| IBIS file bga289.ibs generated by Viper version: 2021.04.12
[IBIS Ver]   5.0
[Comment Char]   |_char
[File Name]   imxrt1180_c0_bga289_consmr.ibs
[File Rev]   1
[Date]   Mon Sep 20 18:29:29 2021
[Source]   NXP Viper 2021.04.12
[Notes]
[Disclaimer] IMPORTANT NOTICE
  This information is provided on an AS IS basis and without warranty.
  IN NO EVENT SHALL NXP BE LIABLE FOR INCIDENTAL OR CONSEQUENTIAL
  DAMAGES ARISING FROM USE OF THIS INFORMATION. THIS DISCLAIMER OF
  WARRANTY EXTENDS TO THE USER OF THE INFORMATION, AND TO THEIR CUSTOMERS
  OR USERS OF PRODUCTS  AND IS IN LIEU OF ALL WARRANTIES WHETHER EXPRESS,
  IMPLIED, OR STATUTORY, INCLUDING IMPLIED WARRANTIES OF MERCHANTABILITY
  OR FITNESS FOR PARTICULAR PURPOSE.
  NXP does not represent or warrant that the information furnished
  hereunder is free of infringement of any third party patents,
  copyrights, trade secrets, or other intellectual property rights.
  NXP does not represent or warrant that the information is free of
  defect, or that it meets any particular standard, requirements or need
  of the user of the infomation or their customers.
  NXP reserves the right to change the information in this file
  without notice.
   http://www.nxp.com
[Copyright]   (C) Copyright NXP 2004 - 2021, All Rights Reserved.
|   BGA289
[Component]   imxrt1180_bga289
[Manufacturer]   NXP
[Package]
| variable   typ   min   max
R_pkg   0.19147   0.066595   0.36415
L_pkg   3.202e-09   1.051e-09   6.257e-09
C_pkg   8.103e-13   6.322e-13   1.390e-12
[Pin] signal_name   model_name   R_pin   L_pin   C_pin
A1   VSS   GND   NA   NA   NA
A2   GPIO_AON_13   FSGPIO   0.33879   6.257e-09 9.609e-13
A3   GPIO_AON_12   FSGPIO   0.31291   5.761e-09 8.893e-13
A4   GPIO_AON_11   FSGPIO   0.29743   5.311e-09 8.120e-13
A5   GPIO_AON_09   FSGPIO   0.28426   5.098e-09 7.847e-13
A6   GPIO_B2_07   STGPIO   0.28355   4.412e-09 7.625e-13
A7   GPIO_B2_08   STGPIO   0.25987   4.038e-09 7.670e-13
A8   GPIO_B2_12   STGPIO   0.23301   4.115e-09 7.409e-13
A9   GPIO_B2_05   STGPIO   0.19229   3.736e-09 7.916e-13
A10   GPIO_B2_10   STGPIO   0.22317   3.759e-09 6.762e-13
A11   GPIO_B1_12   STGPIO   0.23272   3.588e-09 7.397e-13
A12   GPIO_B1_11   STGPIO   0.2418   3.881e-09 7.093e-13
A13   GPIO_B1_10   STGPIO   0.26825   4.052e-09 7.717e-13
A14   GPIO_B1_03   STGPIO   0.23441   4.139e-09 8.811e-13
A15   GPIO_B1_09   STGPIO   0.25617   4.601e-09 8.108e-13
A16   GPIO_SD_B1_05   STGPIO   0.33067   5.525e-09 8.462e-13
A17   VSS   GND   NA   NA   NA
B1   GPIO_AON_08   FSGPIO   0.36415   6.247e-09 9.962e-13
B2   GPIO_AON_14   FSGPIO   0.3511   6.123e-09 9.842e-13
B3   GPIO_AON_15   FSGPIO   0.30751   4.707e-09 1.024e-12
B4   GPIO_AON_04   FSGPIO   0.25099   5.240e-09 8.273e-13
B5   GPIO_AON_10   FSGPIO   0.27824   5.037e-09 7.985e-13
B6   GPIO_AON_02   FSGPIO   0.20191   3.793e-09 8.670e-13
B7   GPIO_AON_01   FSGPIO   0.17543   3.282e-09 7.899e-13
B8   GPIO_B2_13   STGPIO   0.22107   3.526e-09 6.881e-13
B9   GPIO_B2_11   STGPIO   0.19383   3.127e-09 6.881e-13
B10   GPIO_B1_06   STGPIO   0.21843   3.426e-09 7.004e-13
B11   GPIO_B1_13   STGPIO   0.18331   3.168e-09 7.659e-13
B12   GPIO_B1_05   STGPIO   0.18884   3.347e-09 7.743e-13
B13   GPIO_B1_04   STGPIO   0.2248   4.054e-09 8.402e-13
B14   GPIO_B1_08   STGPIO   0.26275   3.772e-09 8.341e-13
B15   GPIO_SD_B1_04   STGPIO   0.26714   3.725e-09 8.042e-13
B16   GPIO_SD_B1_00   STGPIO   0.25592   4.289e-09 8.400e-13
B17   VDD_USB_1P8   POWER   NA   NA   NA
C1   GPIO_AON_24   FSGPIO   0.33893   5.256e-09 9.651e-13
C2   GPIO_AON_23   FSGPIO   0.32781   5.086e-09 1.081e-12
C3   GPIO_AON_22   FSGPIO   0.31081   4.457e-09 1.033e-12
C4   GPIO_AON_26   FSGPIO   0.20352   3.058e-09 8.857e-13
C5   GPIO_AON_16   FSGPIO   0.13111   2.459e-09 1.078e-12
C6   GPIO_AON_07   FSGPIO   0.15435   2.798e-09 1.013e-12
C7   GPIO_AON_05   FSGPIO   0.11787   2.107e-09 9.447e-13
C8   GPIO_AON_03   FSGPIO   0.1131   2.118e-09 9.376e-13
C9   GPIO_B2_04   STGPIO   0.16058   2.823e-09 7.382e-13
C10   GPIO_B2_02   STGPIO   0.14513   2.719e-09 7.407e-13
C11   VSS   GND   NA   NA   NA
C12   GPIO_B1_01   STGPIO   0.14185   2.107e-09 9.331e-13
C13   NVCC_SD1   POWER   NA   NA   NA
C14   VSS   GND   NA   NA   NA
C15   GPIO_SD_B1_03   STGPIO   0.23147   3.505e-09 7.802e-13
C16   USB2_DN   NC   0.24081   4.028e-09 8.124e-13
C17   USB2_DP   NC   0.25149   3.763e-09 8.447e-13
D1   GPIO_EMC_B1_18   STGPIO   0.258   3.820e-09 7.883e-13
D2   GPIO_AON_25   FSGPIO   0.28499   4.052e-09 9.071e-13
D3   GPIO_AON_27   FSGPIO   0.18749   2.960e-09 8.926e-13
D4   VSS   GND   NA   NA   NA
D5   GPIO_AON_19   FSGPIO   0.12727   2.322e-09 8.818e-13
D6   GPIO_AON_17   FSGPIO   0.10329   1.635e-09 9.305e-13
D7   VSS   GND   NA   NA   NA
D8   VSS   GND   NA   NA   NA
D9   GPIO_B2_03   STGPIO   0.11597   1.706e-09 7.096e-13
D10   GPIO_B2_09   STGPIO   0.11311   1.766e-09 7.311e-13
D11   NVCC_GPIO1   POWER   NA   NA   NA
D12   VSS   GND   NA   NA   NA
D13   GPIO_B1_07   STGPIO   0.13862   1.933e-09 9.210e-13
D14   GPIO_SD_B1_02   STGPIO   0.13772   2.370e-09 9.714e-13
D15   GPIO_SD_B1_01   STGPIO   0.15384   2.730e-09 9.985e-13
D16   USB2_VBUS   POWER   0.15839   2.713e-09 9.041e-13
D17   USB1_VBUS   POWER   0.16184   3.951e-09 9.473e-13
E1   GPIO_EMC_B1_09   STGPIO   0.25303   4.125e-09 6.835e-13
E2   GPIO_EMC_B1_17   STGPIO   0.22179   3.357e-09 7.151e-13
E3   GPIO_EMC_B1_10   STGPIO   0.2256   3.189e-09 8.217e-13
E4   GPIO_EMC_B1_29   STGPIO   0.095239  1.607e-09 7.760e-13
E5   GPIO_AON_20   FSGPIO   0.10247   1.686e-09 8.911e-13
E6   GPIO_AON_18   FSGPIO   0.10282   1.671e-09 9.006e-13
E7   GPIO_AON_06   FSGPIO   0.093761  1.482e-09 1.005e-12
E8   GPIO_B2_06   STGPIO   0.1073   1.514e-09 8.020e-13
E9   GPIO_B2_00   STGPIO   0.13841   2.510e-09 7.635e-13
E10   GPIO_B2_01   STGPIO   0.10371   1.433e-09 6.322e-13
E11   NVCC_GPIO1   POWER   NA   NA   NA
E12   GPIO_B1_02   STGPIO   0.1276   2.244e-09 9.489e-13
E13   GPIO_B1_00   STGPIO   0.10548   1.763e-09 9.227e-13
E14   GPIO_SD_B2_07   STGPIO   0.23421   4.029e-09 7.494e-13
E15   GPIO_SD_B2_05   STGPIO   0.18704   3.454e-09 7.592e-13
E16   USB1_DN   NC   0.21779   3.664e-09 9.649e-13
E17   USB1_DP   NC   0.23276   3.528e-09 9.127e-13
F1   GPIO_EMC_B1_23   STGPIO   0.25582   3.688e-09 7.481e-13
F2   GPIO_EMC_B1_11   STGPIO   0.2234   3.528e-09 7.331e-13
F3   GPIO_EMC_B1_13   STGPIO   0.1461   2.557e-09 7.530e-13
F4   GPIO_EMC_B1_19   STGPIO   0.095971  1.490e-09 7.747e-13
F5   GPIO_EMC_B1_28   STGPIO   0.076054  1.222e-09 8.225e-13
F6   GPIO_AON_21   FSGPIO   0.10305   1.731e-09 9.369e-13
F7   NVCC_AON   POWER   NA   NA   NA
F8   GPIO_AON_00   FSGPIO   0.083674  1.456e-09 7.936e-13
F9   NVCC_GPIO2   POWER   NA   NA   NA
F10   NVCC_GPIO2   POWER   NA   NA   NA
F11   VSS   GND   NA   NA   NA
F12   VSS   GND   NA   NA   NA
F13   VSS   GND   NA   NA   NA
F14   GPIO_SD_B2_08   STGPIO   0.22293   3.324e-09 7.483e-13
F15   GPIO_SD_B2_06   STGPIO   0.21283   3.480e-09 7.127e-13
F16   GPIO_SD_B2_09   STGPIO   0.23479   4.008e-09 7.414e-13
F17   GPIO_SD_B2_11   STGPIO   0.26406   4.734e-09 7.048e-13
G1   GPIO_EMC_B1_20   STGPIO   0.2587   4.257e-09 7.360e-13
G2   GPIO_EMC_B1_15   STGPIO   0.21202   2.897e-09 7.576e-13
G3   GPIO_EMC_B1_03   STGPIO   0.11115   2.171e-09 7.587e-13
G4   VSS   GND   NA   NA   NA
G5   GPIO_EMC_B1_14   STGPIO   0.082524  1.274e-09 7.491e-13
G6   GPIO_EMC_B1_12   STGPIO   0.095684  1.724e-09 8.693e-13
G7   VSS   GND   NA   NA   NA
G8   VSS   GND   NA   NA   NA
G9   VSS   GND   NA   NA   NA
G10   VSS   GND   NA   NA   NA
G11   VSS   GND   NA   NA   NA
G12   VDD_USB_3P3   POWER   NA   NA   NA
G13   GPIO_SD_B2_03   STGPIO   0.12063   1.945e-09 7.674e-13
G14   VSS   GND   NA   NA   NA
G15   GPIO_SD_B2_04   STGPIO   0.13723   2.272e-09 8.282e-13
G16   GPIO_SD_B2_10   STGPIO   0.20827   3.251e-09 7.093e-13
G17   GPIO_SD_B2_02   STGPIO   0.24125   3.836e-09 7.672e-13
H1   GPIO_EMC_B1_16   STGPIO   0.24696   4.086e-09 7.264e-13
H2   GPIO_EMC_B1_30   STGPIO   0.20228   2.724e-09 7.288e-13
H3   GPIO_EMC_B1_00   STGPIO   0.11722   2.084e-09 6.738e-13
H4   GPIO_EMC_B1_01   STGPIO   0.11503   2.201e-09 6.863e-13
H5   GPIO_EMC_B1_08   STGPIO   0.081137  1.210e-09 7.720e-13
H6   GPIO_EMC_B1_05   STGPIO   0.11837   2.015e-09 7.999e-13
H7   VSS   GND   NA   NA   NA
H8   VDD_SOC   POWER   NA   NA   NA
H9   VDD_SOC   POWER   NA   NA   NA
H10   VDD_SOC   POWER   NA   NA   NA
H11   VSS   GND   NA   NA   NA
H12   NVCC_SD2   POWER   NA   NA   NA
H13   NVCC_SD2   POWER   NA   NA   NA
H14   GPIO_SD_B2_01   STGPIO   0.11328   2.004e-09 7.188e-13
H15   GPIO_SD_B2_00   STGPIO   0.12994   2.075e-09 7.812e-13
H16   ADC_VREFH   NC   NA   NA   NA
H17   GPIO_AD_35   FSGPIO   0.247   4.250e-09 7.481e-13
J1   GPIO_EMC_B1_32   STGPIO   0.23308   3.732e-09 7.316e-13
J2   GPIO_EMC_B1_31   STGPIO   0.22707   3.554e-09 7.002e-13
J3   GPIO_EMC_B1_27   STGPIO   0.11303   2.145e-09 7.122e-13
J4   GPIO_EMC_B1_04   STGPIO   0.1219   1.967e-09 6.845e-13
J5   NVCC_EMC1   POWER   NA   NA   NA
J6   NVCC_EMC1   POWER   NA   NA   NA
J7   VSS   GND   NA   NA   NA
J8   VDD_SOC   POWER   NA   NA   NA
J9   VDD_SOC   POWER   NA   NA   NA
J10   VDD_SOC   POWER   NA   NA   NA
J11   VSS   GND   NA   NA   NA
J12   DAC_OUT   NC   0.081861  1.217e-09 8.562e-13
J13   VDDA_ADC_1P8   POWER   NA   NA   NA
J14   VDDA_ADC_3P3   POWER   NA   NA   NA
J15   GPIO_AD_34   FSGPIO   0.19425   2.830e-09 6.869e-13
J16   GPIO_AD_33   FSGPIO   0.22403   3.462e-09 7.703e-13
J17   GPIO_AD_32   FSGPIO   0.24678   4.413e-09 6.809e-13
K1   GPIO_EMC_B1_33   STGPIO   0.24584   3.875e-09 7.464e-13
K2   GPIO_EMC_B1_02   STGPIO   0.17777   3.732e-09 7.628e-13
K3   GPIO_EMC_B1_06   STGPIO   0.12968   2.217e-09 7.858e-13
K4   GPIO_EMC_B1_21   STGPIO   0.12677   1.936e-09 7.876e-13
K5   NVCC_EMC1   POWER   NA   NA   NA
K6   DCDC_GND   GND   NA   NA   NA
K7   DCDC_GND   GND   NA   NA   NA
K8   DCDC_GND   GND   NA   NA   NA
K9   DCDC_GND   GND   NA   NA   NA
K10   VDD_SOC   POWER   NA   NA   NA
K11   VSS   GND   NA   NA   NA
K12   GPIO_AD_22   FSGPIO   0.097774  1.685e-09 7.943e-13
K13   GPIO_AD_20   FSGPIO   0.080374  1.560e-09 6.883e-13
K14   GPIO_AD_23   FSGPIO   0.094067  1.530e-09 7.083e-13
K15   GPIO_AD_21   FSGPIO   0.10952   1.994e-09 7.101e-13
K16   GPIO_AD_18   FSGPIO   0.13962   3.133e-09 6.941e-13
K17   GPIO_AD_31   FSGPIO   0.22526   3.913e-09 7.427e-13
L1   GPIO_EMC_B1_35   STGPIO   0.23904   4.022e-09 7.201e-13
L2   GPIO_EMC_B1_34   STGPIO   0.24347   4.235e-09 7.271e-13
L3   GPIO_EMC_B1_22   STGPIO   0.16476   2.932e-09 8.179e-13
L4   VSS   GND   NA   NA   NA
L5   DCDC_PSWITCH   NC   0.17806   2.495e-09 1.035e-12
L6   DCDC_MODE   GND   0.066595  1.051e-09 9.791e-13
L7   DCDC_IN_Q   POWER   0.094007  1.606e-09 9.890e-13
L8   DCDC_SENSE   POWER   0.25313   4.912e-09 1.390e-12
L9   GPIO_BBSM_02   NC   0.12961   2.315e-09 9.450e-13
L10   VSS   GND   NA   NA   NA
L11   VSS   GND   NA   NA   NA
L12   NVCC_GPIO_AD   POWER   NA   NA   NA
L13   GPIO_AD_19   FSGPIO   0.1134   2.198e-09 7.611e-13
L14   VSS   GND   NA   NA   NA
L15   GPIO_AD_29   FSGPIO   0.11504   2.163e-09 6.949e-13
L16   GPIO_AD_28   FSGPIO   0.19564   3.048e-09 6.726e-13
L17   GPIO_AD_30   FSGPIO   0.2232   3.808e-09 6.904e-13
M1   GPIO_EMC_B1_36   STGPIO   0.2659   4.618e-09 7.241e-13
M2   GPIO_EMC_B1_38   STGPIO   0.23883   4.075e-09 8.016e-13
M3   GPIO_EMC_B1_07   STGPIO   0.14046   2.561e-09 8.476e-13
M4   DCDC_1P8   POWER   NA   NA   NA
M5   DCDC_IN   POWER   NA   NA   NA
M6   DCDC_IN   POWER   NA   NA   NA
M7   DCDC_IN   POWER   NA   NA   NA
M8   DCDC_IN   POWER   NA   NA   NA
M9   GPIO_BBSM_06   NC   0.11144   1.997e-09 8.721e-13
M10   GPIO_BBSM_03   NC   0.078718  1.363e-09 8.641e-13
M11   NVCC_GPIO_AD   POWER   NA   NA   NA
M12   VDDA_1P8_IN   POWER   NA   NA   NA
M13   GPIO_AD_24   FSGPIO   0.10138   1.816e-09 7.876e-13
M14   GPIO_AD_26   FSGPIO   0.11318   2.051e-09 7.601e-13
M15   GPIO_AD_25   FSGPIO   0.11488   2.335e-09 7.543e-13
M16   GPIO_AD_27   FSGPIO   0.22269   3.478e-09 7.106e-13
M17   GPIO_AD_17   FSGPIO   0.24535   3.576e-09 7.757e-13
N1   GPIO_EMC_B1_37   STGPIO   0.28475   5.024e-09 7.831e-13
N2   GPIO_EMC_B1_40   STGPIO   0.25351   3.601e-09 8.094e-13
N3   GPIO_EMC_B1_25   STGPIO   0.17316   3.392e-09 9.710e-13
N4   GPIO_EMC_B1_26   STGPIO   0.17245   3.321e-09 1.058e-12
N5   GPIO_EMC_B2_00   STGPIO   0.15819   3.079e-09 9.465e-13
N6   NVCC_EMC2   POWER   NA   NA   NA
N7   NVCC_EMC2   POWER   NA   NA   NA
N8   GPIO_EMC_B2_14   STGPIO   0.074799  1.276e-09 7.132e-13
N9   GPIO_BBSM_08   NC   0.12947   2.224e-09 7.846e-13
N10   GPIO_BBSM_04   NC   0.22225   3.483e-09 8.130e-13
N11   VDDA_1P0   POWER   NA   NA   NA
N12   GPIO_AD_00   FSGPIO   0.10809   1.686e-09 8.787e-13
N13   GPIO_AD_06   FSGPIO   0.08993   1.562e-09 9.011e-13
N14   GPIO_AD_14   FSGPIO   0.11504   2.173e-09 8.152e-13
N15   GPIO_AD_13   FSGPIO   0.1608   2.762e-09 8.198e-13
N16   GPIO_AD_15   FSGPIO   0.161   3.021e-09 7.402e-13
N17   GPIO_AD_16   FSGPIO   0.24707   3.638e-09 7.637e-13
P1   GPIO_EMC_B1_39   STGPIO   0.29637   5.267e-09 7.861e-13
P2   GPIO_EMC_B1_24   STGPIO   0.24228   4.889e-09 8.327e-13
P3   VSS   GND   NA   NA   NA
P4   VSS   GND   NA   NA   NA
P5   GPIO_EMC_B2_02   STGPIO   0.14893   2.798e-09 7.878e-13
P6   GPIO_EMC_B2_11   STGPIO   0.12802   2.133e-09 8.014e-13
P7   VSS   GND   NA   NA   NA
P8   GPIO_EMC_B2_18   STGPIO   0.10803   1.975e-09 7.284e-13
P9   GPIO_BBSM_05   NC   0.11463   1.871e-09 7.041e-13
P10   GPIO_BBSM_01   NC   0.12337   2.055e-09 7.136e-13
P11   VDD_AON_DIG   POWER   NA   NA   NA
P12   VDD_AON_ANA   POWER   NA   NA   NA
P13   GPIO_AD_05   FSGPIO   0.10179   1.883e-09 9.342e-13
P14   VSS   GND   NA   NA   NA
P15   GPIO_AD_04   FSGPIO   0.13812   2.648e-09 8.540e-13
P16   GPIO_AD_11   FSGPIO   0.23441   3.400e-09 7.603e-13
P17   GPIO_AD_12   FSGPIO   0.27648   3.656e-09 7.663e-13
R1   GPIO_EMC_B1_41   STGPIO   0.32006   5.342e-09 8.294e-13
R2   GPIO_EMC_B2_01   STGPIO   0.23332   4.481e-09 8.694e-13
R3   GPIO_EMC_B2_04   STGPIO   0.24846   3.983e-09 7.214e-13
R4   GPIO_EMC_B2_15   STGPIO   0.21336   2.929e-09 7.975e-13
R5   GPIO_EMC_B2_12   STGPIO   0.17332   3.366e-09 7.727e-13
R6   GPIO_EMC_B2_13   STGPIO   0.1322   2.415e-09 7.678e-13
R7   GPIO_EMC_B2_16   STGPIO   0.12695   2.303e-09 7.485e-13
R8   GPIO_EMC_B2_20   STGPIO   0.19566   2.797e-09 7.446e-13
R9   GPIO_BBSM_07   NC   0.12219   1.958e-09 6.935e-13
R10   GPIO_BBSM_00   NC   0.18852   2.914e-09 6.903e-13
R11   GPIO_BBSM_09   NC   0.21079   3.399e-09 6.774e-13
R12   VDD_BBSM_ANA   POWER   NA   NA   NA
R13   GPIO_AD_02   FSGPIO   0.11226   2.074e-09 9.819e-13
R14   GPIO_AD_01   FSGPIO   0.14525   2.746e-09 9.176e-13
R15   GPIO_AD_03   FSGPIO   0.16734   3.237e-09 9.293e-13
R16   GPIO_AD_09   FSGPIO   0.23818   3.983e-09 8.801e-13
R17   GPIO_AD_10   FSGPIO   0.25673   4.696e-09 7.060e-13
T1   DCDC_LP   POWER   NA   NA   NA
T2   DCDC_LP   POWER   NA   NA   NA
T3   DCDC_LP   POWER   NA   NA   NA
T4   GPIO_EMC_B2_05   STGPIO   0.27282   4.100e-09 7.178e-13
T5   GPIO_EMC_B2_03   STGPIO   0.23231   3.470e-09 7.245e-13
T6   GPIO_EMC_B2_06   STGPIO   0.20608   3.243e-09 7.148e-13
T7   GPIO_EMC_B2_07   STGPIO   0.15363   3.064e-09 6.931e-13
T8   WAKEUP   NC   0.20117   3.201e-09 7.461e-13
T9   PMIC_STBY_REQ   NC   0.19408   3.132e-09 7.980e-13
T10   POR_B   NC   0.22023   3.727e-09 7.387e-13
T11   TEST_MODE   NC   0.2307   4.062e-09 7.020e-13
T12   VSS   GND   NA   NA   NA
T13   RTC_XTALI   NC   0.20768   3.768e-09 8.695e-13
T14   GPIO_AD_08   FSGPIO   0.22481   3.670e-09 9.400e-13
T15   CLK1_N   NC   0.29048   4.443e-09 8.625e-13
T16   XTALO   NC   0.27619   4.750e-09 9.551e-13
T17   GPIO_AD_07   FSGPIO   0.29195   5.173e-09 8.895e-13
U1   VSS   GND   NA   NA   NA
U2   DCDC_LP   POWER   NA   NA   NA
U3   DCDC_LP   POWER   NA   NA   NA
U4   GPIO_EMC_B2_08   STGPIO   0.28328   4.128e-09 7.323e-13
U5   GPIO_EMC_B2_09   STGPIO   0.25203   4.385e-09 7.783e-13
U6   GPIO_EMC_B2_10   STGPIO   0.21486   3.751e-09 7.837e-13
U7   GPIO_EMC_B2_17   STGPIO   0.24417   3.583e-09 7.307e-13
U8   GPIO_EMC_B2_19   STGPIO   0.25689   3.714e-09 7.525e-13
U9   PMIC_ON_REQ   NC   0.23427   4.038e-09 7.305e-13
U10   ONOFF   NC   0.24002   4.183e-09 7.492e-13
U11   NVCC_BBSM   POWER   NA   NA   NA
U12   VDD_BBSM_IN   POWER   NA   NA   NA
U13   RTC_XTALO   NC   0.21404   3.930e-09 8.574e-13
U14   VDD_AON_IN   POWER   NA   NA   NA
U15   CLK1_P   NC   0.29899   4.254e-09 8.645e-13
U16   XTALI   NC   0.28595   4.814e-09 1.003e-12
U17   VSS   GND   NA   NA   NA
[Pin Mapping]   pulldown_ref   pullup_ref
A1   VSS   NC
A2   VSS   NVCC_AON
A3   VSS   NVCC_AON
A4   VSS   NVCC_AON
A5   VSS   NVCC_AON
A6   VSS   NVCC_GPIO2
A7   VSS   NVCC_GPIO2
A8   VSS   NVCC_GPIO2
A9   VSS   NVCC_GPIO2
A10   VSS   NVCC_GPIO2
A11   VSS   NVCC_GPIO1
A12   VSS   NVCC_GPIO1
A13   VSS   NVCC_GPIO1
A14   VSS   NVCC_GPIO1
A15   VSS   NVCC_GPIO1
A16   VSS   NVCC_SD1
A17   VSS   NC
B1   VSS   NVCC_AON
B2   VSS   NVCC_AON
B3   VSS   NVCC_AON
B4   VSS   NVCC_AON
B5   VSS   NVCC_AON
B6   VSS   NVCC_AON
B7   VSS   NVCC_AON
B8   VSS   NVCC_GPIO2
B9   VSS   NVCC_GPIO2
B10   VSS   NVCC_GPIO1
B11   VSS   NVCC_GPIO1
B12   VSS   NVCC_GPIO1
B13   VSS   NVCC_GPIO1
B14   VSS   NVCC_GPIO1
B15   VSS   NVCC_SD1
B16   VSS   NVCC_SD1
B17   NC   VDD_USB_1P8
C1   VSS   NVCC_AON
C2   VSS   NVCC_AON
C3   VSS   NVCC_AON
C4   VSS   NVCC_AON
C5   VSS   NVCC_AON
C6   VSS   NVCC_AON
C7   VSS   NVCC_AON
C8   VSS   NVCC_AON
C9   VSS   NVCC_GPIO2
C10   VSS   NVCC_GPIO2
C11   VSS   NC
C12   VSS   NVCC_GPIO1
C13   NC   NVCC_SD1
C14   VSS   NC
C15   VSS   NVCC_SD1
C16   NC   NC
C17   NC   NC
D1   VSS   NVCC_EMC1
D2   VSS   NVCC_AON
D3   VSS   NVCC_AON
D4   VSS   NC
D5   VSS   NVCC_AON
D6   VSS   NVCC_AON
D7   VSS   NC
D8   VSS   NC
D9   VSS   NVCC_GPIO2
D10   VSS   NVCC_GPIO2
D11   NC   NVCC_GPIO1
D12   VSS   NC
D13   VSS   NVCC_GPIO1
D14   VSS   NVCC_SD1
D15   VSS   NVCC_SD1
D16   NC   VDD_USB_3P3
D17   NC   VDD_USB_3P3
E1   VSS   NVCC_EMC1
E2   VSS   NVCC_EMC1
E3   VSS   NVCC_EMC1
E4   VSS   NVCC_EMC1
E5   VSS   NVCC_AON
E6   VSS   NVCC_AON
E7   VSS   NVCC_AON
E8   VSS   NVCC_GPIO2
E9   VSS   NVCC_GPIO2
E10   VSS   NVCC_GPIO2
E11   NC   NVCC_GPIO1
E12   VSS   NVCC_GPIO1
E13   VSS   NVCC_GPIO1
E14   VSS   NVCC_SD2
E15   VSS   NVCC_SD2
E16   NC   NC
E17   NC   NC
F1   VSS   NVCC_EMC1
F2   VSS   NVCC_EMC1
F3   VSS   NVCC_EMC1
F4   VSS   NVCC_EMC1
F5   VSS   NVCC_EMC1
F6   VSS   NVCC_AON
F7   NC   NVCC_AON
F8   VSS   NVCC_AON
F9   NC   NVCC_GPIO2
F10   NC   NVCC_GPIO2
F11   VSS   NC
F12   VSS   NC
F13   VSS   NC
F14   VSS   NVCC_SD2
F15   VSS   NVCC_SD2
F16   VSS   NVCC_SD2
F17   VSS   NVCC_SD2
G1   VSS   NVCC_EMC1
G2   VSS   NVCC_EMC1
G3   VSS   NVCC_EMC1
G4   VSS   NC
G5   VSS   NVCC_EMC1
G6   VSS   NVCC_EMC1
G7   VSS   NC
G8   VSS   NC
G9   VSS   NC
G10   VSS   NC
G11   VSS   NC
G12   NC   VDD_USB_3P3
G13   VSS   NVCC_SD2
G14   VSS   NC
G15   VSS   NVCC_SD2
G16   VSS   NVCC_SD2
G17   VSS   NVCC_SD2
H1   VSS   NVCC_EMC1
H2   VSS   NVCC_EMC1
H3   VSS   NVCC_EMC1
H4   VSS   NVCC_EMC1
H5   VSS   NVCC_EMC1
H6   VSS   NVCC_EMC1
H7   VSS   NC
H8   NC   VDD_SOC
H9   NC   VDD_SOC
H10   NC   VDD_SOC
H11   VSS   NC
H12   NC   NVCC_SD2
H13   NC   NVCC_SD2
H14   VSS   NVCC_SD2
H15   VSS   NVCC_SD2
H16   NC   NC
H17   VSS   NVCC_GPIO_AD
J1   VSS   NVCC_EMC1
J2   VSS   NVCC_EMC1
J3   VSS   NVCC_EMC1
J4   VSS   NVCC_EMC1
J5   NC   NVCC_EMC1
J6   NC   NVCC_EMC1
J7   VSS   NC
J8   NC   VDD_SOC
J9   NC   VDD_SOC
J10   NC   VDD_SOC
J11   VSS   NC
J12   NC   NC
J13   NC   VDDA_ADC_1P8
J14   NC   VDDA_ADC_3P3
J15   VSS   NVCC_GPIO_AD
J16   VSS   NVCC_GPIO_AD
J17   VSS   NVCC_GPIO_AD
K1   VSS   NVCC_EMC1
K2   VSS   NVCC_EMC1
K3   VSS   NVCC_EMC1
K4   VSS   NVCC_EMC1
K5   NC   NVCC_EMC1
K6   DCDC_GND   NC
K7   DCDC_GND   NC
K8   DCDC_GND   NC
K9   DCDC_GND   NC
K10   NC   VDD_SOC
K11   VSS   NC
K12   VSS   NVCC_GPIO_AD
K13   VSS   NVCC_GPIO_AD
K14   VSS   NVCC_GPIO_AD
K15   VSS   NVCC_GPIO_AD
K16   VSS   NVCC_GPIO_AD
K17   VSS   NVCC_GPIO_AD
L1   VSS   NVCC_EMC1
L2   VSS   NVCC_EMC1
L3   VSS   NVCC_EMC1
L4   VSS   NC
L5   NC   NC
L6   DCDC_MODE   NC
L7   NC   DCDC_IN_Q
L8   NC   DCDC_SENSE
L9   NC   NC
L10   VSS   NC
L11   VSS   NC
L12   NC   NVCC_GPIO_AD
L13   VSS   NVCC_GPIO_AD
L14   VSS   NC
L15   VSS   NVCC_GPIO_AD
L16   VSS   NVCC_GPIO_AD
L17   VSS   NVCC_GPIO_AD
M1   VSS   NVCC_EMC1
M2   VSS   NVCC_EMC1
M3   VSS   NVCC_EMC1
M4   NC   DCDC_1P8
M5   NC   DCDC_IN
M6   NC   DCDC_IN
M7   NC   DCDC_IN
M8   NC   DCDC_IN
M9   NC   NC
M10   NC   NC
M11   NC   NVCC_GPIO_AD
M12   NC   VDDA_1P8_IN
M13   VSS   NVCC_GPIO_AD
M14   VSS   NVCC_GPIO_AD
M15   VSS   NVCC_GPIO_AD
M16   VSS   NVCC_GPIO_AD
M17   VSS   NVCC_GPIO_AD
N1   VSS   NVCC_EMC1
N2   VSS   NVCC_EMC1
N3   VSS   NVCC_EMC1
N4   VSS   NVCC_EMC1
N5   VSS   NVCC_EMC2
N6   NC   NVCC_EMC2
N7   NC   NVCC_EMC2
N8   VSS   NVCC_EMC2
N9   NC   NC
N10   NC   NC
N11   NC   VDDA_1P0
N12   VSS   NVCC_GPIO_AD
N13   VSS   NVCC_GPIO_AD
N14   VSS   NVCC_GPIO_AD
N15   VSS   NVCC_GPIO_AD
N16   VSS   NVCC_GPIO_AD
N17   VSS   NVCC_GPIO_AD
P1   VSS   NVCC_EMC1
P2   VSS   NVCC_EMC1
P3   VSS   NC
P4   VSS   NC
P5   VSS   NVCC_EMC2
P6   VSS   NVCC_EMC2
P7   VSS   NC
P8   VSS   NVCC_EMC2
P9   NC   NC
P10   NC   NC
P11   NC   VDD_AON_DIG
P12   NC   VDD_AON_ANA
P13   VSS   NVCC_GPIO_AD
P14   VSS   NC
P15   VSS   NVCC_GPIO_AD
P16   VSS   NVCC_GPIO_AD
P17   VSS   NVCC_GPIO_AD
R1   VSS   NVCC_EMC1
R2   VSS   NVCC_EMC2
R3   VSS   NVCC_EMC2
R4   VSS   NVCC_EMC2
R5   VSS   NVCC_EMC2
R6   VSS   NVCC_EMC2
R7   VSS   NVCC_EMC2
R8   VSS   NVCC_EMC2
R9   NC   NC
R10   NC   NC
R11   NC   NC
R12   NC   VDD_BBSM_ANA
R13   VSS   NVCC_GPIO_AD
R14   VSS   NVCC_GPIO_AD
R15   VSS   NVCC_GPIO_AD
R16   VSS   NVCC_GPIO_AD
R17   VSS   NVCC_GPIO_AD
T1   NC   DCDC_LP
T2   NC   DCDC_LP
T3   NC   DCDC_LP
T4   VSS   NVCC_EMC2
T5   VSS   NVCC_EMC2
T6   VSS   NVCC_EMC2
T7   VSS   NVCC_EMC2
T8   NC   NC
T9   NC   NC
T10   NC   NC
T11   NC   NC
T12   VSS   NC
T13   NC   NC
T14   VSS   NVCC_GPIO_AD
T15   NC   NC
T16   NC   NC
T17   VSS   NVCC_GPIO_AD
U1   VSS   NC
U2   NC   DCDC_LP
U3   NC   DCDC_LP
U4   VSS   NVCC_EMC2
U5   VSS   NVCC_EMC2
U6   VSS   NVCC_EMC2
U7   VSS   NVCC_EMC2
U8   VSS   NVCC_EMC2
U9   NC   NC
U10   NC   NC
U11   NC   NVCC_BBSM
U12   NC   VDD_BBSM_IN
U13   NC   NC
U14   NC   VDD_AON_IN
U15   NC   NC
U16   NC   NC
U17   VSS   NC
|*   Model Selector   *
[Model Selector] STGPIO
BDPROGSCARUDQP_SDMMC_3V3SF_00_SD   PSW=0 High Drive, 1V8 SD
BDPROGSCARUDQP_SDMMC_3V3SF_01_SD   PSW=0 Low Drive,  1V8 SD
BDPROGSCARUDQP_SDMMC_3V3SF_00_MMC   PSW=0 High Drive, 1V8 MMC
BDPROGSCARUDQP_SDMMC_3V3SF_01_MMC   PSW=0 Low Drive,  1V8 MMC
BDPROGSCARUDQP_SDMMC_3V3SF_10   PSW=1 High Drive, 3V3 +/- 10%, SD & 3V3 MMC
BDPROGSCARUDQP_SDMMC_3V3SF_11   PSW=1 Low Drive,  3V3 +/- 10%, SD & 3V3 MMC
BDPROGSCARUDQP_SDMMC_3V3SF_10_5pct  PSW=1 High Drive, 3V3 +/- 5%, SD & 3V3 MMC
BDPROGSCARUDQP_SDMMC_3V3SF_11_5pct  PSW=1 Low Drive,  3V3 +/- 5%, SD & 3V3 MMC
BDPROGSCARUDQP_SDMMC_3V3SF_11_2v7   PSW=1 Low Drive,  2V7 SD & 2V7 MMC
BDPROGSCARUDQP_SDMMC_3V3SF_10_2v7   PSW=1 High Drive, 2V7 SD & 2V7 MMC
[Model Selector] FSGPIO
io_crnrobe1dse0sre0   Normal range in cont mode, 5mA drive strength, without slew rate
io_crnrobe1dse0sre1   Normal range in cont mode, 5mA drive strength, with slew rate
io_crnrobe1dse1sre0   Normal range in cont mode, 10mA drive strength, without slew rate
io_crnrobe1dse1sre1   Normal range in cont mode, 10mA drive strength, with slew rate
io_crdrobe1dse0sre0   Derated range in cont mode, 5mA drive strength, without slew rate
io_crdrobe1dse0sre1   Derated range in cont mode, 5mA drive strength, with slew rate
io_crdrobe1dse1sre0   Derated range in cont mode, 10mA drive strength, without slew rate
io_crdrobe1dse1sre1   Derated range in cont mode, 10mA drive strength, with slew rate
io_crdr2obe1dse0sre0   Derated2 range in cont mode, 5mA drive strength, without slew rate
io_crdr2obe1dse0sre1   Derated2 range in cont mode, 5mA drive strength, with slew rate
io_crdr2obe1dse1sre0   Derated2 range in cont mode, 10mA drive strength, without slew rate
io_crdr2obe1dse1sre1   Derated2 range in cont mode, 10mA drive strength, with slew rate
io_hrobe1dse0sre0   high range mode, 5mA drive strength, without slew rate
io_hrobe1dse0sre1   high range mode, 5mA drive strength, with slew rate
io_hrobe1dse1sre0   high range mode, 10mA drive strength, without slew rate
io_hrobe1dse1sre1   high range mode, 10mA drive strength, with slew rate
io_lrobe1dse0sre0   low range mode, 5mA drive strength, without slew rate
io_lrobe1dse0sre1   low range mode, 5mA drive strength, with slew rate
io_lrobe1dse1sre0   low range mode, 10mA drive strength, without slew rate
io_lrobe1dse1sre1   low range mode, 10mA drive strength, with slew rate
io_crnrobe1dse0sre0_5pct   Narrow range in cont mode, 5mA drive strength, without slew rate
io_crnrobe1dse0sre1_5pct   Narrow range in cont mode, 5mA drive strength, with slew rate
io_crnrobe1dse1sre0_5pct   Narrow range in cont mode, 10mA drive strength, without slew rate
io_crnrobe1dse1sre1_5pct   Narrow range in cont mode, 10mA drive strength, with slew rate
io_hrobe1dse0sre0_5pct   Narrow range in high range mode, 5mA drive strength, without slew rate
io_hrobe1dse0sre1_5pct   Narrow range in high range mode, 5mA drive strength, with slew rate
io_hrobe1dse1sre0_5pct   Narrow range in high range mode, 10mA drive strength, without slew rate
io_hrobe1dse1sre1_5pct   Narrow range in high range mode, 10mA drive strength, with slew rate
|End  [Component] imxrt1180_bga289
| Models and submodels in the file (38): BDPROGSCARUDQP_SDMMC_3V3SF_00_MMC (I/O), BDPROGSCARUDQP_SDMMC_3V3SF_00_SD (I/O), BDPROGSCARUDQP_SDMMC_3V3SF_01_MMC (I/O), BDPROGSCARUDQP_SDMMC_3V3SF_01_SD (I/O), BDPROGSCARUDQP_SDMMC_3V3SF_10 (I/O), BDPROGSCARUDQP_SDMMC_3V3SF_11 (I/O), BDPROGSCARUDQP_SDMMC_3V3SF_10_2v7 (I/O), BDPROGSCARUDQP_SDMMC_3V3SF_11_2v7 (I/O), BDPROGSCARUDQP_SDMMC_3V3SF_10_5pct (I/O), BDPROGSCARUDQP_SDMMC_3V3SF_11_5pct (I/O), io_crnrobe1dse0sre0 (I/O), io_crnrobe1dse0sre1 (I/O), io_crnrobe1dse1sre0 (I/O), io_crnrobe1dse1sre1 (I/O), io_crdrobe1dse0sre0 (I/O), io_crdrobe1dse0sre1 (I/O), io_crdrobe1dse1sre0 (I/O), io_crdrobe1dse1sre1 (I/O), io_crdr2obe1dse0sre0 (I/O), io_crdr2obe1dse0sre1 (I/O), io_crdr2obe1dse1sre0 (I/O), io_crdr2obe1dse1sre1 (I/O), io_hrobe1dse0sre0 (I/O), io_hrobe1dse0sre1 (I/O), io_hrobe1dse1sre0 (I/O), io_hrobe1dse1sre1 (I/O), io_lrobe1dse0sre0 (I/O), io_lrobe1dse0sre1 (I/O), io_lrobe1dse1sre0 (I/O), io_lrobe1dse1sre1 (I/O), io_crnrobe1dse0sre0_5pct (I/O), io_crnrobe1dse0sre1_5pct (I/O), io_crnrobe1dse1sre0_5pct (I/O), io_crnrobe1dse1sre1_5pct (I/O), io_hrobe1dse0sre0_5pct (I/O), io_hrobe1dse0sre1_5pct (I/O), io_hrobe1dse1sre0_5pct (I/O), io_hrobe1dse1sre1_5pct (I/O)
